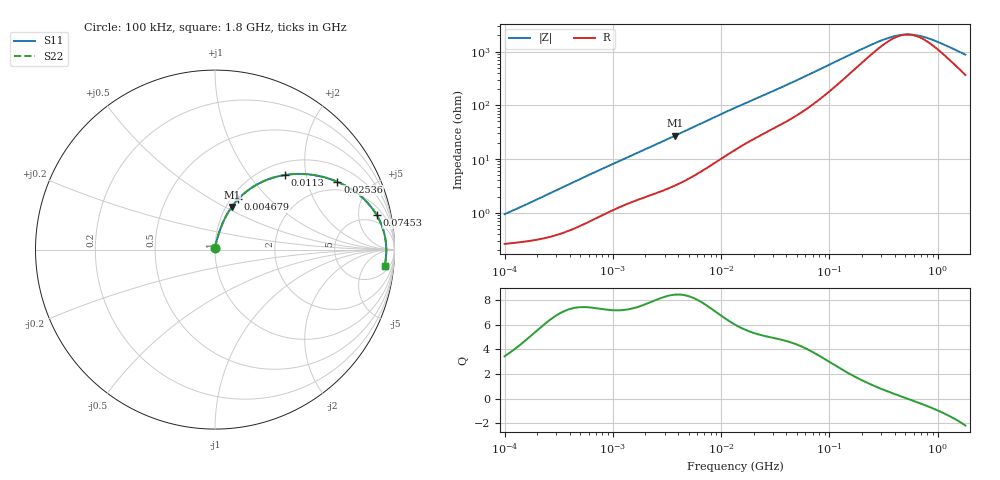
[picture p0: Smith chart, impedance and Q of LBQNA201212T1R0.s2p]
! LBQNA201212T1R0  S-PARAMETER MODEL  ( General Type )
! Model Generated by TAIYO YUDEN Corporation (http://www.ty-top.com)
! Version 1.0
! TAIYO YUDEN Control No. 191025NI43SB-FBB
! Copyright(c) 2019 TAIYO YUDEN CO.,LTD. All Rights Reserved.
! Product Description (link to TY-COMPAS)
! https://ds.yuden.co.jp/TYCOMPAS/or/detail?pn=LBQNA201212T1R0M&u=M
! Products Name : Inductors
! Characteristics :
!  Inductance : 1.0 uH , SRF(min) : 100 MHz , DC Resistance(max) : 0.195 Ohm
!  Rated Current : Saturation :500 mA , Temp Rise : 700 mA (20 degC)
!  Case Size : 2.0 x 1.25 / 0.079 x 0.049 [mm/inch] , Thickness : 1.25 / 0.049 [mm/inch]
!  (Conditions: Temperature = 25 degC , DC Bias Current/Voltage = 0A / 0V)
! External Node Assignments :
!  1  o---GGG---o  2
! GND o---------o GND
! Frequency Range : 0.1MHz  -  1800MHz  [ 402 STEP ]
# MHz S RI R 50
! Freq[MHz].  S11 Real  S11 Imag  S21 Real  S21 Imag  S12 Real  S12 Imag  S22 Real  S22 Imag
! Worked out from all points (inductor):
!   401 points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, 100 kHz to 1.8 GHz, reference 50 ohm
!   read as one part in series: L = 1.41 uH near 105 kHz
!   highest Q = 8.44 at 3.754 MHz (marker M1), where L = 1.15 uH
!   self-resonance near 525.8 MHz
!   S11 on the Smith chart (normalised r, x): 100 kHz: 1.01, +0.02; 4.679 MHz: 1.08, +0.67; 11.3 MHz: 1.24, +1.52; 25.36 MHz: 1.61, +3.10; 74.53 MHz: 3.27, +8.29; 1.8 GHz: 8, -16
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0.1  0.00269 0.00899  0.9973 -0.00899  0.9973 -0.00899  0.00269 0.00899
0.155413  0.00308 0.0136  0.9969 -0.0136  0.9969 -0.0136  0.00308 0.0136
0.516129  0.00767 0.0429  0.9923 -0.0429  0.9923 -0.0429  0.00767 0.0429
1.277529  0.0231 0.0962  0.9769 -0.0962  0.9769 -0.0962  0.0231 0.0962
2.66389  0.0581 0.1802  0.9419 -0.1802  0.9419 -0.1802  0.0581 0.1802
3.753625  0.0936 0.238  0.9064 -0.238  0.9064 -0.238  0.0936 0.238
4.679446  0.1284 0.2802  0.8716 -0.2802  0.8716 -0.2802  0.1284 0.2802
7.096489  0.2281 0.3593  0.7719 -0.3593  0.7719 -0.3593  0.2281 0.3593
11.30236  0.3886 0.4157  0.6114 -0.4157  0.6114 -0.4157  0.3886 0.4157
13.41641  0.4542 0.4216  0.5458 -0.4216  0.5458 -0.4216  0.4542 0.4216
18.00091  0.565 0.4128  0.435 -0.4128  0.435 -0.4128  0.565 0.4128
25.36465  0.6821 0.3776  0.3179 -0.3776  0.3179 -0.3776  0.6821 0.3776
41.39926  0.8124 0.2973  0.1876 -0.2973  0.1876 -0.2973  0.8124 0.2973
69.24595  0.8942 0.2031  0.1058 -0.2031  0.1058 -0.2031  0.8942 0.2031
74.52619  0.9018 0.1906  0.0982 -0.1906  0.0982 -0.1906  0.9018 0.1906
151.6408  0.942 0.0937  0.058 -0.0937  0.058 -0.0937  0.942 0.0937
259.9299  0.9512 0.0457  0.0488 -0.0457  0.0488 -0.0457  0.9512 0.0457
357.3983  0.9534 0.0237  0.0466 -0.0237  0.0466 -0.0237  0.9534 0.0237
491.4156  0.9542 0.00406  0.0458 -0.00406  0.0458 -0.00406  0.9542 0.00406
675.6865  0.9541 -0.0153  0.0459 0.0153  0.0459 0.0153  0.9541 -0.0153
952.0939  0.953 -0.0378  0.047 0.0378  0.047 0.0378  0.953 -0.0378
1800  0.9453 -0.0933  0.0547 0.0933  0.0547 0.0933  0.9453 -0.0933
